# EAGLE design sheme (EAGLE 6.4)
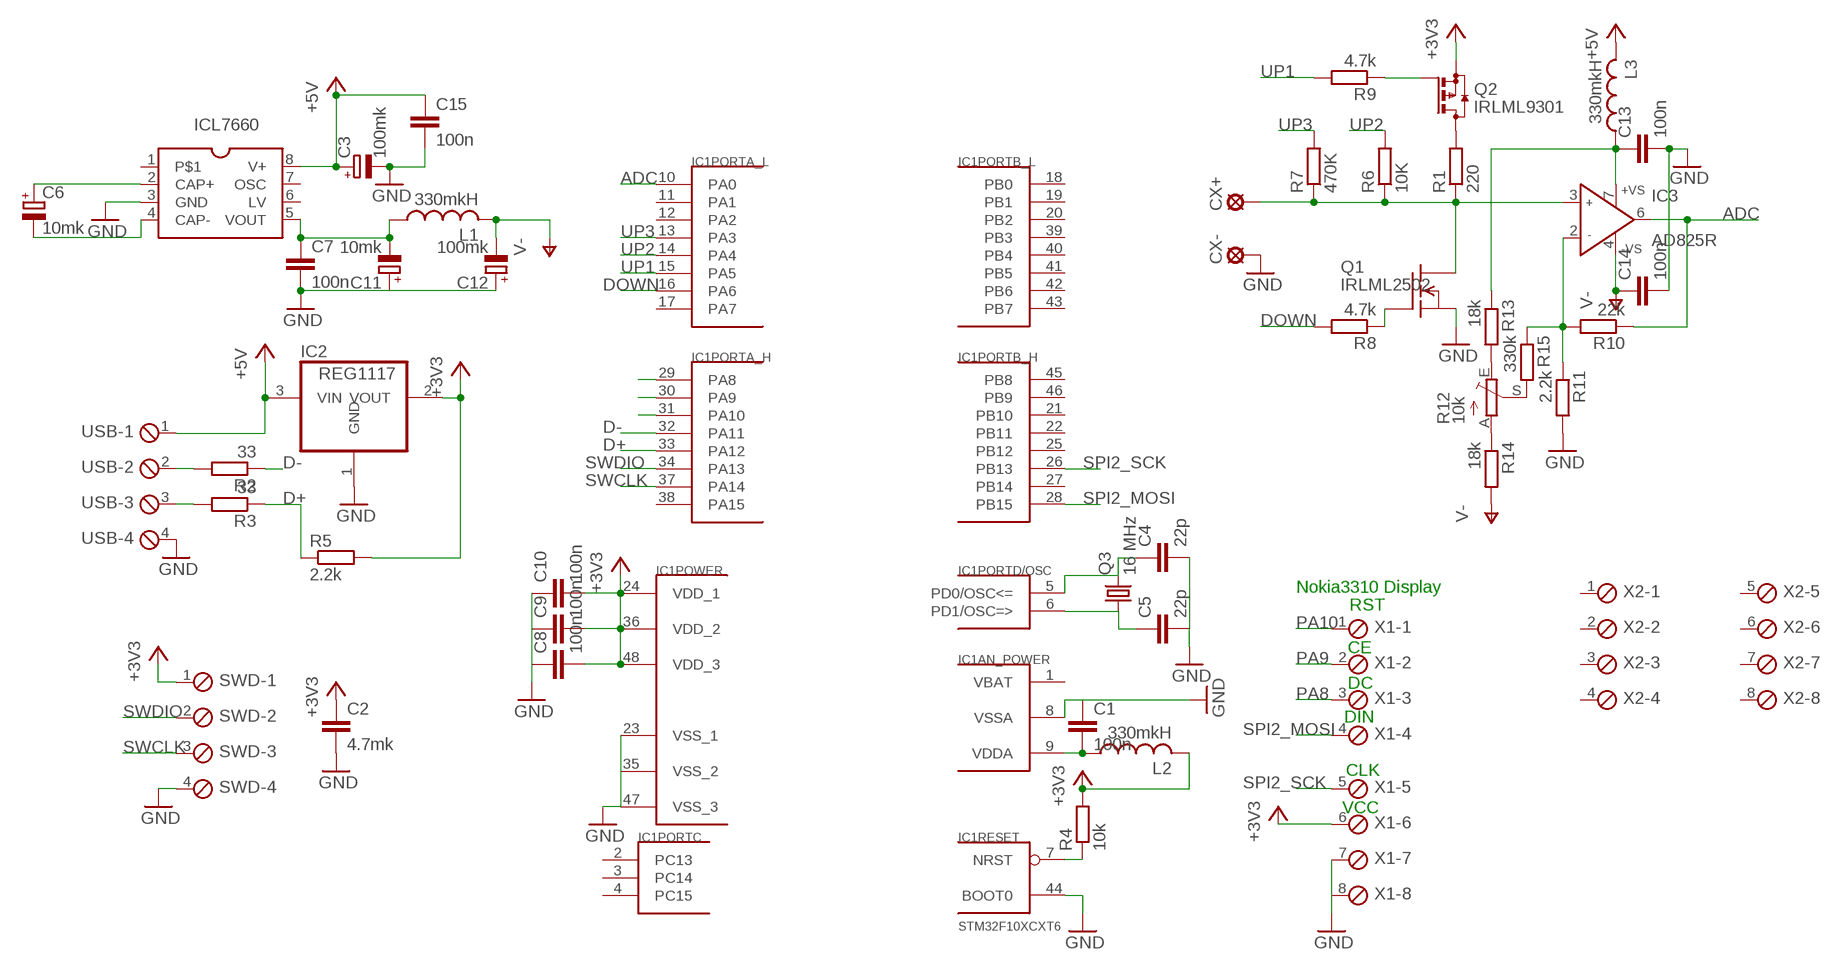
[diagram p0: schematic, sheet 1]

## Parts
C1  100n  C-EUC0805  [C0805]
C2  4.7mk  C-EUC0805  [C0805]
C3  100mk  CPOL-EUE2,5-6E  [E2,5-6E]
C4  22p  C-EUC0805  [C0805]
C5  22p  C-EUC0805  [C0805]
C6  10mk  CPOL-EUE2,5-6E  [E2,5-6E]
C7  100n  C-EUC0805  [C0805]
C8  100n  C-EUC0805  [C0805]
C9  100n  C-EUC0805  [C0805]
C10  100n  C-EUC0805  [C0805]
C11  10mk  CPOL-EUE2,5-6E  [E2,5-6E]
C12  100mk  CPOL-EUE2,5-6E  [E2,5-6E]
C13  100n  C-EUC0805  [C0805]
C14  100n  C-EUC0805  [C0805]
C15  100n  C-EUC0805  [C0805]
CX+  SE14  [SE14]
CX-  SE14  [SE14]
IC1  STM32F10XCXT6  [TQFP48]
IC2  REG1117  [SOT223]
IC3  AD825R  [SO8]
ICL7660  ICL7660  [SO8]
L1  330mkH  L-US0204/7  [0204/7]
L2  330mkH  L-US0204/7  [0204/7]
L3  330mkH  L-US0204/7  [0204/7]
Q1  IRLML2502  [SOT23]
Q2  IRLML9301  BSS84  [SOT23]
Q3  16 MHz  CRYSTALHC49S  [HC49/S]
R1  220  R-EU_M0805  [M0805]
R2  33  R-EU_R1206W  [R1206W]
R3  33  R-EU_R1206W  [R1206W]
R4  10k  R-EU_M0805  [M0805]
R5  2.2k  R-EU_M0805  [M0805]
R6  10K  R-EU_M0805  [M0805]
R7  470K  R-EU_M0805  [M0805]
R8  4.7k  R-EU_M0805  [M0805]
R9  4.7k  R-EU_M0805  [M0805]
R10  22k  R-EU_M0805  [M0805]
R11  2.2k  R-EU_M0805  [M0805]
R12  10k  TRIM_EU-RJ9W  [RJ9W]
R13  18k  R-EU_M0805  [M0805]
R14  18k  R-EU_M0805  [M0805]
R15  330k  R-EU_M0805  [M0805]
SWD  MPT4  [4POL254]
USB  MPT4  [4POL254]
X1  MPT8  [8POL254]
X2  MPT8  [8POL254]

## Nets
+3V3: C2.1 C8.2 C9.2 C10.2 IC1.24(POWER:VDD_1) IC1.36(POWER:VDD_2) IC1.48(POWER:VDD_3) IC2.2(VOUT) L2.2 Q2.2(S) R4.2 R5.2 SWD.1 X1.6
+5V: C3.+ C15.1 IC2.3(VIN) ICL7660.8(V+) L3.2 USB.1
ADC: IC1.10(PORTA_L:PA0) IC3.6(OUT) R10.1
D+: IC1.33(PORTA_H:PA12) R3.1 R5.1
D-: IC1.32(PORTA_H:PA11) R2.1
DOWN: IC1.16(PORTA_L:PA6) R8.2
GND: C1.1 C2.2 C3.- C4.2 C5.2 C7.2 C8.1 C9.1 C10.1 C11.+ C12.+ C13.2 C14.2 C15.2 CX-.MP IC1.8(AN_POWER:VSSA) IC1.23(POWER:VSS_1) IC1.35(POWER:VSS_2) IC1.44(RESET:BOOT0) IC1.47(POWER:VSS_3) IC2.1(GND) ICL7660.3(GND) Q1.2(S) R11.2 SWD.4 USB.4 X1.7 X1.8
N$1: C4.1 IC1.5(PORTD/OSC:PD0/OSC<=) Q3.2
N$2: C5.1 IC1.6(PORTD/OSC:PD1/OSC=>) Q3.1
N$3: C6.+ ICL7660.2(CAP+)
N$4: R2.2 USB.2
N$5: R3.2 USB.3
N$6: Q2.3(D) R1.2
N$7: CX+.MP IC3.3(IN+) Q1.3(D) R1.1 R6.1 R7.1
N$8: Q1.1(G) R8.1
N$9: C6.- ICL7660.4(CAP-)
N$10: C13.1 IC3.7(+VS) L3.1 R13.1
N$11: R12.S R15.2
N$12: Q2.1(G) R9.1
N$13: R12.E R13.2
N$14: R12.A R14.1
N$15: IC1.7(RESET:NRST) R4.1
N$16: C1.2 IC1.9(AN_POWER:VDDA) L2.1
N$17: IC3.2(IN-) R10.2 R11.1 R15.1
N$18: C7.1 C11.- ICL7660.5(VOUT) L1.1
PA8: IC1.29(PORTA_H:PA8) X1.3
PA9: IC1.30(PORTA_H:PA9) X1.2
PA10: IC1.31(PORTA_H:PA10) X1.1
SPI2_MOSI: IC1.28(PORTB_H:PB15) X1.4
SPI2_SCK: IC1.26(PORTB_H:PB13) X1.5
SWCLK: IC1.37(PORTA_H:PA14) SWD.3
SWDIO: IC1.34(PORTA_H:PA13) SWD.2
UP1: IC1.15(PORTA_L:PA5) R9.2
UP2: IC1.14(PORTA_L:PA4) R6.2
UP3: IC1.13(PORTA_L:PA3) R7.2
V-: C12.- C14.1 IC3.4(-VS) L1.2 R14.2
Unconnected: IC1.2(PORTC:PC13) IC1.3(PORTC:PC14) IC1.4(PORTC:PC15) IC1.11(PORTA_L:PA1) IC1.12(PORTA_L:PA2) IC1.17(PORTA_L:PA7) IC1.18(PORTB_L:PB0) IC1.19(PORTB_L:PB1) IC1.20(PORTB_L:PB2) IC1.21(PORTB_H:PB10) IC1.22(PORTB_H:PB11) IC1.25(PORTB_H:PB12) IC1.27(PORTB_H:PB14) IC1.38(PORTA_H:PA15) IC1.39(PORTB_L:PB3) IC1.40(PORTB_L:PB4) IC1.41(PORTB_L:PB5) IC1.42(PORTB_L:PB6) IC1.43(PORTB_L:PB7) IC1.45(PORTB_H:PB8) IC1.46(PORTB_H:PB9) ICL7660.1 ICL7660.6(LV) ICL7660.7(OSC) X2.1 X2.2 X2.3 X2.4 X2.5 X2.6 X2.7 X2.8

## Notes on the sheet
- ICL7660
- Nokia3310 Display
- RST
- CE
- DC
- DIN
- CLK
- VCC

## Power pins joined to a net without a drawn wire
VBAT: IC1.1(AN_POWER:VBAT)

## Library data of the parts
C1 C2 C4 C5 C7-C10 C13-C15 = resistor:C-EU: CAPACITOR, European symbol
C3 C6 C11 C12 = rcl:CPOL-EU: POLARIZED CAPACITOR, European symbol
CX+ CX- = solpad:SE14: SOLDER PAD
IC1 = stm32:STM32F10XCXT6: ST STM32F101/103 48pin LQFP
IC2 = burr-brown:REG1117: 800mA and 1A Low Dropout (LDO) Positive Regulator 1.8V, 2.5V, 2.85V, 3.3V, 5V, and Adj; MPN: REG1117; OC_FARNELL: 1097566; OC_NEWARK: 14P6981
IC3 = analog-devices:AD825: Low Cost, General-Purpose High Speed JFET Amplifier Source: http://www.analog.com/static/imported-files/data_sheets/AD825.pdf; MF: ALTERA CORPORATION; MPN: AD825ARZ; OC_FARNELL: 9603735; OC_NEWARK: 59K6528
ICL7660 = balmer:ICL7660
L1-L3 = rcl:L-US: INDUCTOR, American symbol
Q1 = balmer:IRLML2502
Q2 = transistor-small-signal:BSS84: P-CHANNEL MOS FET
Q3 = crystal:CRYSTAL: CRYSTAL; OC_FARNELL: 1667008; OC_NEWARK: unknown
R1-R11 R13-R15 = rcl:R-EU_: RESISTOR, European symbol
R12 = pot:TRIM_EU-: POTENTIOMETER
SWD USB = con-phoenix-254:MPT4: PHOENIX CONNECTOR; OC_FARNELL: unknown; OC_NEWARK: unknown
X1 X2 = con-phoenix-254:MPT8: PHOENIX CONNECTOR; OC_FARNELL: unknown; OC_NEWARK: unknown

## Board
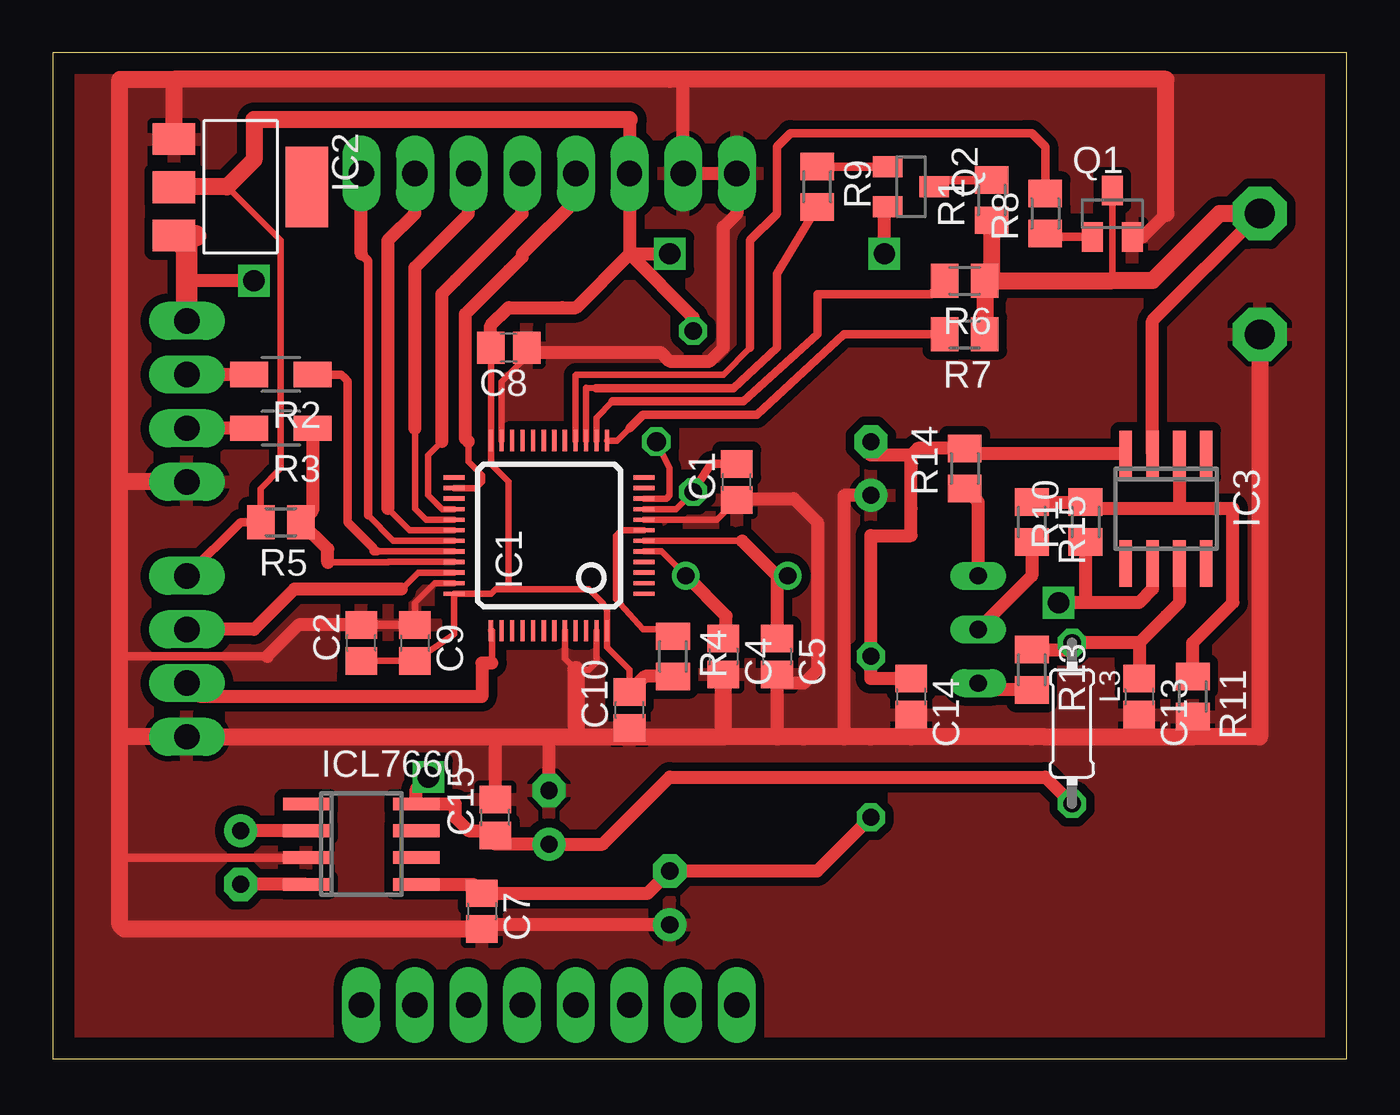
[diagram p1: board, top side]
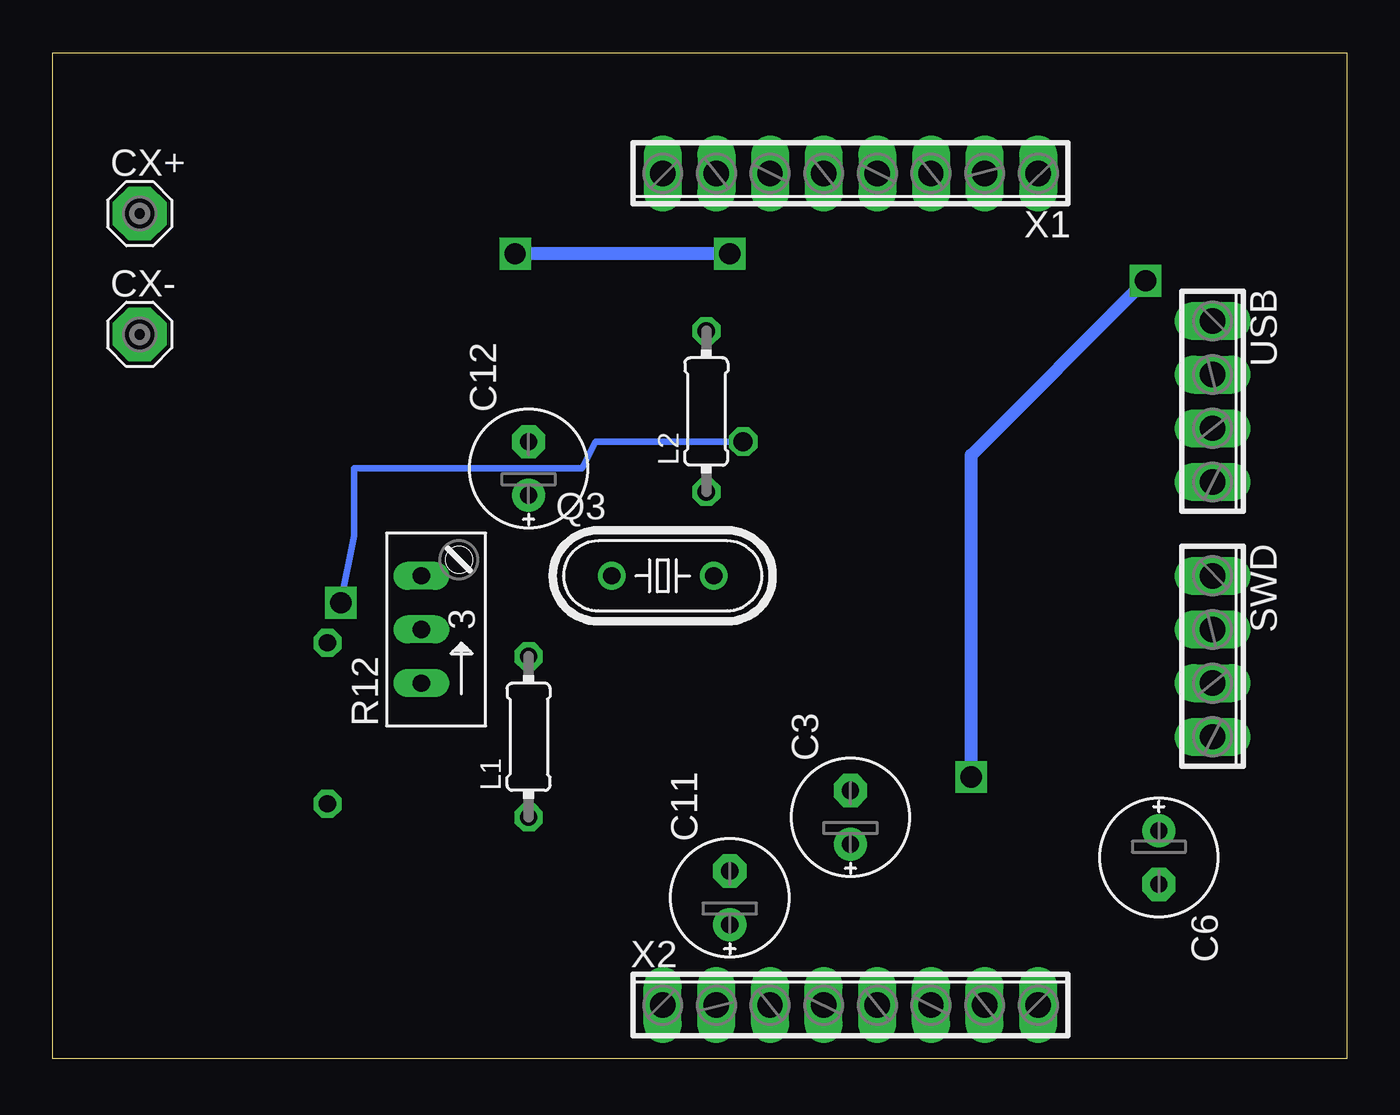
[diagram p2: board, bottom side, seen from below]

Size 61.27 x 47.62 mm. Coordinates in mm from the lower left corner, seen from the top.
Outline: 0,0 61.27,0 61.27,47.62 0,47.62 0,0
Copper layers (1*16): Top 0.035mm / dielectric 1.5mm / Bottom 0.035mm
Design rules "default": minimum track width 10mil, minimum drill 24mil, track to track 8mil, track to pad 8mil, pad to pad 8mil, via to via 8mil, smd to smd 8mil, copper to edge 40mil, drill to drill 8mil, minimum pad ring 10mil, minimum via ring 8mil, stop-mask expansion 4mil, vias tented up to drill 0mil, thermal gap 10mil

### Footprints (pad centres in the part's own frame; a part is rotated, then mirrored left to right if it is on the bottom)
C0805 = smd 1.3 x 1.5: 1 -0.85,0; 2 0.85,0
E2,5-6E = drill 0.813 pad 1.575: + -1.27,0 | drill 0.813 pad 1.575 octagon: - 1.27,0
SE14 = drill 1.397 pad 2.54 octagon: MP 0,0
TQFP48 = smd 0.2 x 1: 1 -2.75,-4.5; 2 -2.25,-4.5; 3 -1.75,-4.5; 4 -1.25,-4.5; 5 -0.75,-4.5; 6 -0.25,-4.5; 7 0.25,-4.5; 8 0.75,-4.5; 9 1.25,-4.5; 10 1.75,-4.5; 11 2.25,-4.5; 12 2.75,-4.5; 25 2.75,4.5; 26 2.25,4.5; 27 1.75,4.5; 28 1.25,4.5; 29 0.75,4.5; 30 0.25,4.5; 31 -0.25,4.5; 32 -0.75,4.5; 33 -1.25,4.5; 34 -1.75,4.5; 35 -2.25,4.5; 36 -2.75,4.5 | smd 1 x 0.2: 13 4.5,-2.75; 14 4.5,-2.25; 15 4.5,-1.75; 16 4.5,-1.25; 17 4.5,-0.75; 18 4.5,-0.25; 19 4.5,0.25; 20 4.5,0.75; 21 4.5,1.25; 22 4.5,1.75; 23 4.5,2.25; 24 4.5,2.75; 37 -4.5,2.75; 38 -4.5,2.25; 39 -4.5,1.75; 40 -4.5,1.25; 41 -4.5,0.75; 42 -4.5,0.25; 43 -4.5,-0.25; 44 -4.5,-0.75; 45 -4.5,-1.25; 46 -4.5,-1.75; 47 -4.5,-2.25; 48 -4.5,-2.75
SOT223 = smd 1.499 x 2.007: 1 -2.261,-3.15; 2 0.025,-3.15; 3 2.311,-3.15 | smd 3.81 x 2.007: 4 0,3.15
SO8 = smd 0.6 x 2.2: 1 -1.905,-2.6; 2 -0.635,-2.6; 3 0.635,-2.6; 4 1.905,-2.6; 5 1.905,2.6; 6 0.635,2.6; 7 -0.635,2.6; 8 -1.905,2.6
0204/7 = drill 0.813 octagon: 1 -3.81,0; 2 3.81,0
SOT23 = smd 1 x 1.4: 1 -0.95,-1.1; 2 0.95,-1.1; 3 0,1.1
HC49/S = drill 0.813: 1 -2.413,0; 2 2.413,0
M0805 = smd 1.3 x 1.6: 1 -0.95,0; 2 0.95,0
R1206W = smd 1.8 x 1.2: 1 -1.499,0; 2 1.499,0
RJ9W = drill 0.813 long: A 2.54,0.635; E -2.54,0.635; S 0,0.635
4POL254 = drill 1.2 long: 1 -3.81,0; 2 -1.27,0; 3 1.27,0; 4 3.81,0
8POL254 = drill 1.2 long: 1 -8.89,0; 2 -6.35,0; 3 -3.81,0; 4 -1.27,0; 5 1.27,0; 6 3.81,0; 7 6.35,0; 8 8.89,0

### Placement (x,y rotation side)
C1  32.38,27.3 90 top
C2  14.61,19.68 90 top
C3  23.5,11.43 90 bottom
C4  31.75,19.05 270 top
C5  34.29,19.05 270 top
C6  8.89,9.53 270 bottom
C7  20.32,6.99 270 top
C8  21.59,33.66 180 top
C9  17.14,19.68 270 top
C10  27.3,16.51 90 top
C11  29.21,7.62 90 bottom
C12  38.73,27.94 90 bottom
C13  51.44,17.14 270 top
C14  40.64,17.14 270 top
C15  20.95,11.43 90 top
CX+  57.15,40.01 0 bottom
CX-  57.15,34.29 0 bottom
IC1  23.5,24.77 90 top
IC2  8.89,41.27 270 top
IC3  52.7,26.04 180 top
ICL7660  14.61,10.16 270 top
L1  38.73,15.24 90 bottom
L2  30.32,30.64 90 bottom
L3  48.26,15.88 270 top
Q1  50.16,40.01 0 top
Q2  40.64,41.27 270 top
Q3  32.38,22.86 0 bottom
R1  44.45,40.64 90 top
R2  10.79,32.38 180 top
R3  10.79,29.84 180 top
R4  29.37,19.05 270 top
R5  10.79,25.4 180 top
R6  43.18,36.83 180 top
R7  43.18,34.29 180 top
R8  46.99,40.01 90 top
R9  36.2,41.27 270 top
R10  48.9,25.4 90 top
R11  53.98,17.14 270 top
R12  43.18,20.32 90 bottom
R13  46.35,18.41 270 top
R14  43.18,27.94 90 top
R15  46.35,25.4 270 top
SWD  6.35,19.05 270 bottom
USB  6.35,31.11 270 bottom
X1  23.5,41.91 180 bottom
X2  23.5,2.54 0 bottom

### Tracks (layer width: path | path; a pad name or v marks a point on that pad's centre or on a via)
+3V3  (via drill 1)
  Top 0.305: C2.1 C9.2 19,20.11 IC1.36 20.75,22.02 20.95,22.23 21.59,22.23 | 21.59,22.23 25.4,22.23 26.04,21.59 26.25,21.22 IC1.48 26.25,19.48 27.3,18.41 C10.2 | C8.2 20.75,30.05 20.75,29.84 IC1.24 20.75,28.15 21.59,27.3 21.59,22.23 | R5.2 9.85,26.99 10.79,27.94 10.79,38.73 8.26,41.27
  Top 0.406: R5.2 8.89,25.4 SWD.1
  Top 0.61: R4.2 28.05,18.1 C10.2 | C8.2 20.74,34.71 21.59,35.56 24.13,35.56 24.77,35.56 27.3,38.1 | 27.3,44.45 X1.6 27.3,38.1 | 27.3,38.1 v29.21,38.1 | L2.2 30.32,35.08 27.3,38.1 | v39.37,38.1 39.37,40.16 Q2.2
  Top 0.813: 27.3,44.45 9.53,44.45 9.53,42.55 8.26,41.27 5.77,41.27 IC2.2
  Bottom 0.61: v29.21,38.1 v39.37,38.1
+5V  (via drill 1)
  Top 0.61: v17.78,13.34 17.2,12.76 ICL7660.8 19.05,12.06 19.05,11.43 19.68,10.79 20.74,10.79 C15.1 20.95,10.16 C3.+ 26.04,10.16 29.21,13.34 46.99,13.34 L3.2 | v9.53,36.83 6.35,36.83
  Top 1.016: 6.76,38.96 IC2.3 6.35,38.35 6.35,36.83 USB.1
  Bottom 0.61: v17.78,13.34 17.78,28.57 v9.53,36.83
ADC  (via drill 0.9, 1)
  Top 0.305: IC1.10 28.42,26.52 29.05,26.52 29.21,26.67 29.21,27.3 29.21,27.94 v28.57,29.21
  Top 0.61: IC3.6 52.07,22.23 51.44,21.59 48.9,21.59 | 48.9,21.59 v47.62,21.59 | R10.1 48.9,21.59
  Bottom 0.305: v47.62,21.59 46.99,24.77 46.99,27.94 36.2,27.94 35.56,29.21 v28.57,29.21
D+
  Top 0.305: IC1.33 15.89,23.52 15.88,23.5 13.02,23.5
  Top 0.61: 13.02,23.5 13.02,24.13 R5.1 12.29,25.95 R3.1
D-
  Top 0.305: IC1.32 15.36,24.02
  Top 0.406: R2.1 13.65,32.38 13.81,32.23 13.97,32.07 13.97,25.4 15.2,24.17 15.2,24.02 15.36,24.02
DOWN
  Top 0.305: IC1.16 24.75,32.37 24.77,32.38 31.75,32.38 33.02,33.66
  Top 0.406: 33.02,33.66 33.02,38.73 34.29,40.01 34.29,43.18 34.92,43.81 46.04,43.81 46.35,43.81 46.99,43.18 R8.2
GND
  Top 0.305: C1.1 31.45,25.52 IC1.8 | IC1.47 25.75,18.76 25.4,18.41 24.77,18.41 24.25,18.93 IC1.44 | C10.1 27.3,15.24 | IC1.35 18.07,22.52 17.14,21.59 C9.1 | IC1.23 21.25,32.04 22.23,33.02 22.23,33.44 | 22.23,33.44 C8.1 22.23,33.44
  Top 0.406: C2.2 C9.1 | 10.16,19.05 3.17,19.05 | ICL7660.3 3.17,9.53
  Top 0.61: C2.2 11.64,20.54 10.16,19.05 | C1.1 32.44,26.51 35.08,26.51 36.2,25.4 36.2,18.41 35.56,17.78 34.71,17.78 C5.2 34.29,15.24 | C13.2 51.44,15.24 | 22.23,33.44 28.79,33.44 29.21,33.02 31.11,33.02 31.75,33.66 31.75,34.29 31.75,36.83 31.75,39.37 32.38,40.01 X1.8 X1.7 29.84,46.35 | R11.2 53.98,15.24 | C14.2 40.64,15.24 | C12.+ 37.47,26.67 37.47,15.24 | C3.- 23.5,15.24 | C15.2 20.95,15.24 | C11.+ 20.54,6.35 C7.2 | Q1.2 51.6,38.91 52.7,40.01
  Top 0.813: 24.77,15.24 23.5,15.24 20.95,15.24 SWD.4 3.17,15.24 | 24.77,15.24 27.3,15.24 31.75,15.24 | 31.75,15.24 C4.2 | 24.77,18.41 24.77,15.24 | 31.75,15.24 34.29,15.24 35.56,15.24 37.47,15.24 38.73,15.24 40.64,15.24 46.35,15.24 46.99,15.24 51.44,15.24 53.98,15.24 57.15,15.24 CX-.MP | 5.71,46.35 29.21,46.35 29.84,46.35 52.7,46.35 52.7,40.01 | IC2.1 5.74,46.33 5.71,46.35 | 3.17,15.24 3.17,19.05 3.17,27.3 | 3.17,27.3 3.17,46.35 5.71,46.35 | USB.4 3.17,27.3 | C7.2 3.39,6.13 3.17,6.35 3.17,9.53 3.17,15.24
  pour Top (isolate 0.406): 0,0 0,47.62 60.96,47.62 60.96,0
N$1
  Top 0.305: IC1.5 28.82,24.02 Q3.2
  Top 0.61: C4.1 31.88,20.03 31.88,20.95 Q3.2
N$2
  Top 0.305: IC1.6 32.63,24.52
  Top 0.61: Q3.1 34.29,22.86 | 34.29,22.86 32.63,24.52 | 34.29,22.86 C5.1
N$3
  Top 0.61: ICL7660.2 C6.+
N$4
  Top 0.61: R2.2 USB.2
N$5
  Top 0.61: R3.2 USB.3
N$6
  Top 0.406: R1.2 42.05,41.59 Q2.3
N$7
  Top 0.305: Q1.3 50.16,36.83
  Top 0.61: IC3.3 52.07,34.92 CX+.MP
  Top 0.813: R1.1 44.45,37.15 R6.1 | R6.1 R7.1 | R6.1 50.16,36.83 52.07,36.83 55.24,40.01 CX+.MP
N$8
  Top 0.406: Q1.1 47.14,38.91 R8.1
N$9
  Top 0.61: ICL7660.4 C6.-
N$10
  Top 0.61: 51.44,19.68 52.7,20.95 53.34,21.59 IC3.7 | 51.44,19.68 C13.1 | 51.44,19.68 L3.1 47.94,19.36 R13.1
N$11
  Top 0.61: R15.2 46.35,22.86 R12.S
N$12
  Top 0.406: R9.1 Q2.1
N$13
  Top 0.61: R13.2 44.13,17.46 R12.E
N$14
  Top 0.61: R12.A 43.81,26.36 R14.1
N$15
  Top 0.305: IC1.7 26.92,25.02 26.67,24.77 26.67,22.23 26.67,21.91 26.67,21.75 27.94,20.32 28.89,20.32 R4.1
N$16
  Top 0.305: IC1.9 29.03,26.02 29.51,26.02 L2.1
  Top 0.406: C1.2 31.17,28.16 L2.1
N$17
  Top 0.61: R15.1 R10.2 49.21,26.04 53.34,26.04 | R11.1 53.98,19.68 55.88,21.59 55.88,26.04 53.34,26.04 | IC3.2 53.34,26.04
N$18
  Top 0.61: ICL7660.5 19.9,8.26 C7.1 28.16,7.83 C11.- 36.2,8.89 L1.1
PA8
  Top 0.305: IC1.29 17.66,25.52 17.14,26.04 17.14,29.84
  Top 0.61: 17.14,29.84 17.14,37.47 19.68,40.01 X1.3
PA9
  Top 0.305: IC1.30 16.89,25.02 15.88,26.04
  Top 0.61: 15.88,26.04 15.88,38.73 17.14,40.01 X1.2
PA10
  Top 0.305: IC1.31 16.12,24.52 14.92,25.72
  Top 0.406: 14.92,25.72 14.92,37.78 14.61,38.1
  Top 0.61: 14.61,38.1 X1.1
SPI2_MOSI
  Top 0.305: IC1.28 18.43,26.02 17.78,26.67 17.78,28.57 18.41,29.21
  Top 0.61: 18.41,29.21 18.41,36.2 19.05,36.83 22.23,40.01 X1.4
SPI2_SCK
  Top 0.305: IC1.26 20.03,27.02 20.32,27.3 20.32,27.62 19.68,28.26 19.68,29.21
  Top 0.61: 19.68,29.21 19.53,29.37 19.53,35.24 21.59,37.31 22.23,37.94 22.23,38.1 24.77,40.64 X1.5
SWCLK
  Top 0.305: IC1.37 20.8,20.27 20.8,18.73
  Top 0.61: 20.8,18.73 20.32,18.73 20.32,17.14 6.99,17.14 SWD.3
SWDIO
  Top 0.305: IC1.34 17.3,23.02 16.51,22.23
  Top 0.61: 16.51,22.23 11.43,22.23 9.53,20.32 SWD.2
UP1
  Top 0.305: IC1.15 25.25,31.75 25.72,31.75
  Top 0.406: 25.72,31.75 32.23,31.75 34.29,33.66 34.29,37.15 R9.2
UP2
  Top 0.305: IC1.14 25.75,30.19 25.75,30.35 26.51,31.11
  Top 0.406: 26.51,31.11 32.7,31.11 36.2,34.29 36.2,36.2 41.59,36.2 R6.2
UP3
  Top 0.305: IC1.13 26.73,29.27 27.3,29.84
  Top 0.406: 27.3,29.84 27.94,30.48 33.34,30.48 37.47,34.29 R7.2
V-
  Top 0.61: C14.1 38.73,18 L1.2 38.73,24.77 40.64,24.77 40.64,26.04 40.64,27.94 | 40.64,27.94 40.64,28.57 | 40.64,28.57 38.73,28.57 C12.- | 40.64,28.25 40.64,27.94 | 40.64,28.57 40.95,28.89 R14.2 43.44,28.64 IC3.4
